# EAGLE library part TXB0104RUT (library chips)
4-channel bidirectional level translater
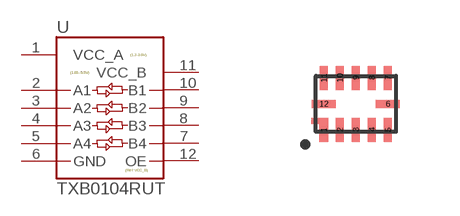
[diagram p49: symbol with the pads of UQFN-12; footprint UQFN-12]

Designator prefix U

## TXB0104RUT (DIGIKEY: 296-25888-1-ND; MANUFACTURER: TI; MPN: TXB0104RUTR)  [UQFN-12]
1  VCC_A
2  A1
3  A2
4  A3
5  A4
6  GND
7  B4
8  B3
9  B2
10  B1
11  VCC_B
12  OE

## Footprint UQFN-12 (pad centres in mm)
smd 0.2 x 0.6: 1 -0.8,-0.65; 2 -0.4,-0.65; 3 0,-0.65; 4 0.4,-0.65; 5 0.8,-0.65; 7 0.8,0.65; 8 0.4,0.65; 9 0,0.65; 10 -0.4,0.65; 11 -0.8,0.65
smd 0.6 x 0.2: 6 0.8,0; 12 -0.8,0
